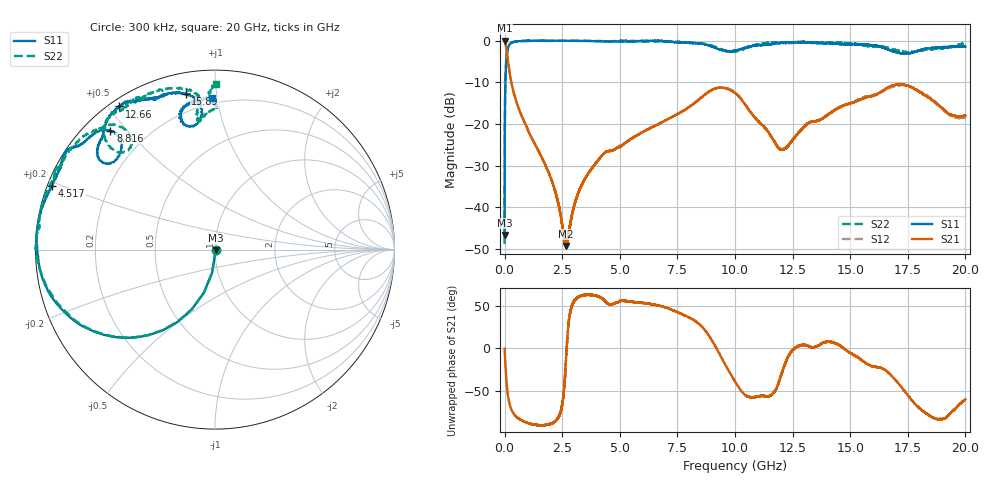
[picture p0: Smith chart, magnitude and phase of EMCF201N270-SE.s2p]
!EMCF201N270
!Johanson Technology Inc.
!www.johansontechnology.com
!Test Board Conditions:
!Substrate Type  RO4350B
!Substrate Thickness  6.6 mil
!Substrate Dk  3.66
!TL Type: GCPW
!TL Trace Width  13 mil
!TL Gap  7.5 mil
!PART MODE SINGLE ENDED (AKA BYPASS)
!DUT TOPOLOGY	SERIES-SHUNT
# MHz S  dB  R 50
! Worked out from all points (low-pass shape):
!   20001 points, 300 kHz to 20 GHz, reference 50 ohm
!   highest |S21| = 0.01 dB at 300 kHz (marker M1); lowest = -49.3 dB at 2.678 GHz (marker M2)
!   |S21| within 3 dB of the highest: start of sweep to 99.99 MHz
!   lowest |S11| = -46.7 dB at 300 kHz (marker M3), VSWR 1.01, Z = 50.4 - j0.236 ohm
!   |S11| at or under -10 dB: start of sweep to 34.13 MHz
!   |S22| runs from -48.8 to 0.0 dB; largest |S21 - S12| = 0.011
!   S11 on the Smith chart (normalised r, x): 300 kHz: 1.01, -0.00; 4.517 GHz: 0.01, +0.19; 8.816 GHz: 0.07, +0.45; 12.66 GHz: 0.03, +0.53; 15.89 GHz: 0.11, +0.82; 20 GHz: 0.16, +0.96
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0.3  -46.66 -30.3  0.01 -0.4  0.02 -0.4  -48.79 -19.1
104.298  -2.95 -136.3  -3.18 -46.1  -3.15 -46.0  -3.00 -136.3
213.297  -0.91 -156.2  -7.67 -65.3  -7.63 -65.4  -0.97 -156.7
457.293  -0.24 -169.7  -13.71 -79.0  -13.70 -79.2  -0.24 -170.8
1100.284  -0.09 -178.2  -22.53 -88.8  -22.56 -88.5  -0.02 176.7
2070.269  -0.03 172.6  -33.97 -88.4  -33.93 -88.3  -0.11 172.8
2678.26  -0.04 168.1  -49.34 -7.2  -49.05 -7.4  -0.06 169.6
3334.25  -0.08 165.4  -34.86 62.0  -34.83 62.0  -0.03 164.1
4517.232  -0.22 158.5  -26.52 52.0  -26.54 52.2  -0.17 156.3
6667.2  -0.07 146.2  -20.08 50.6  -20.04 50.3  -0.15 147.4
8816.168  -1.08 131.3  -12.48 16.9  -12.53 17.1  -0.93 128.9
10000.15  -2.44 140.6  -12.59 -39.0  -12.41 -38.6  -2.65 132.5
10930.14  -1.16 138.1  -18.92 -56.9  -18.98 -57.8  -0.99 133.9
11936.12  -0.60 130.2  -26.02 -37.0  -25.97 -36.3  -0.51 125.9
12660.11  -0.37 123.7  -22.82 1.6  -22.66 1.2  -0.47 120.6
13334.1  -0.50 119.3  -19.50 1.4  -19.39 1.0  -0.56 116.1
15885.06  -1.10 100.7  -13.37 -20.3  -13.23 -21.5  -1.35 96.2
16667.05  -2.20 95.5  -11.17 -28.7  -11.47 -29.4  -1.79 96.5
17405.04  -3.08 100.6  -10.71 -51.9  -10.74 -50.7  -2.75 97.4
18174.03  -2.12 103.9  -12.92 -74.0  -12.67 -73.6  -2.29 92.2
19295.01  -1.51 96.6  -17.65 -78.0  -17.71 -80.1  -1.58 91.1
20000  -1.44 91.3  -18.01 -60.0  -18.39 -58.9  -0.68 89.5
